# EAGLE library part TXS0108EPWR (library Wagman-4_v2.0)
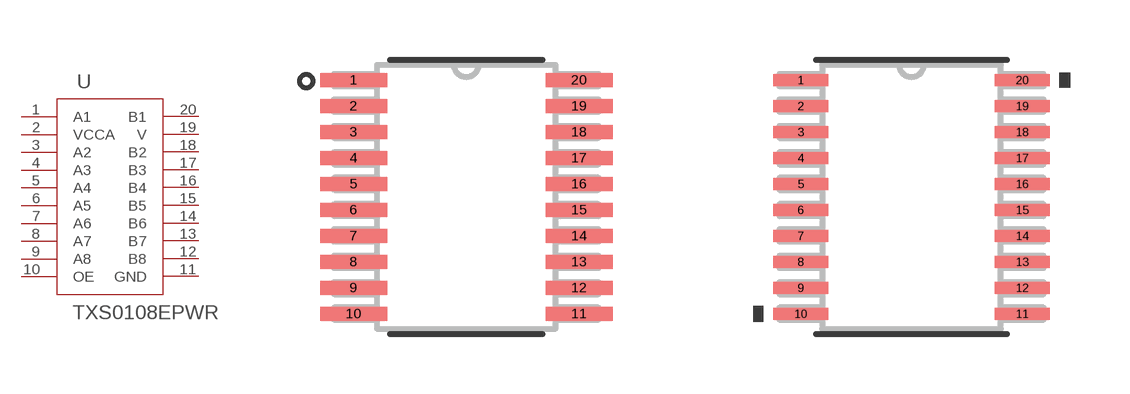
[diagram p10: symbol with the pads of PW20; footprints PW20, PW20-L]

Designator prefix U

## TXS0108EPWR (MANUFACTURER_PART_NUMBER: TXS0108EPWR; VENDOR: Texas Instruments)  [PW20]
1  A1
2  VCCA  pwr
3  A2
4  A3
5  A4
6  A5
7  A6
8  A7
9  A8
10  OE  out
11  GND  pwr
12  B8
13  B7
14  B6
15  B5
16  B4
17  B3
18  B2
19  V  pwr
20  B1

## TXS0108EPWRPW20-L (MANUFACTURER_PART_NUMBER: TXS0108EPWR; VENDOR: Texas Instruments)  [PW20-L]
Pads as for PW20

## TXS0108EPWRPW20-M (MANUFACTURER_PART_NUMBER: TXS0108EPWR; VENDOR: Texas Instruments)  [PW20-M]
Pads as for PW20

## Footprint PW20 (pad centres in mm)
smd 1.676 x 0.356: 1 -2.819,2.925; 2 -2.819,2.275; 3 -2.819,1.625; 4 -2.819,0.975; 5 -2.819,0.325; 6 -2.819,-0.325; 7 -2.819,-0.975; 8 -2.819,-1.625; 9 -2.819,-2.275; 10 -2.819,-2.925; 11 2.819,-2.925; 12 2.819,-2.275; 13 2.819,-1.625; 14 2.819,-0.975; 15 2.819,-0.325; 16 2.819,0.325; 17 2.819,0.975; 18 2.819,1.625; 19 2.819,2.275; 20 2.819,2.925

## Footprint PW20-L (pad centres in mm)
smd 1.372 x 0.305: 1 -2.769,2.925; 2 -2.769,2.275; 3 -2.769,1.625; 4 -2.769,0.975; 5 -2.769,0.325; 6 -2.769,-0.325; 7 -2.769,-0.975; 8 -2.769,-1.625; 9 -2.769,-2.275; 10 -2.769,-2.925; 11 2.769,-2.925; 12 2.769,-2.275; 13 2.769,-1.625; 14 2.769,-0.975; 15 2.769,-0.325; 16 2.769,0.325; 17 2.769,0.975; 18 2.769,1.625; 19 2.769,2.275; 20 2.769,2.925

## Footprint PW20-M (pad centres in mm)
smd 1.981 x 0.406: 1 -2.87,2.925; 2 -2.87,2.275; 3 -2.87,1.625; 4 -2.87,0.975; 5 -2.87,0.325; 6 -2.87,-0.325; 7 -2.87,-0.975; 8 -2.87,-1.625; 9 -2.87,-2.275; 10 -2.87,-2.925; 11 2.87,-2.925; 12 2.87,-2.275; 13 2.87,-1.625; 14 2.87,-0.975; 15 2.87,-0.325; 16 2.87,0.325; 17 2.87,0.975; 18 2.87,1.625; 19 2.87,2.275; 20 2.87,2.925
